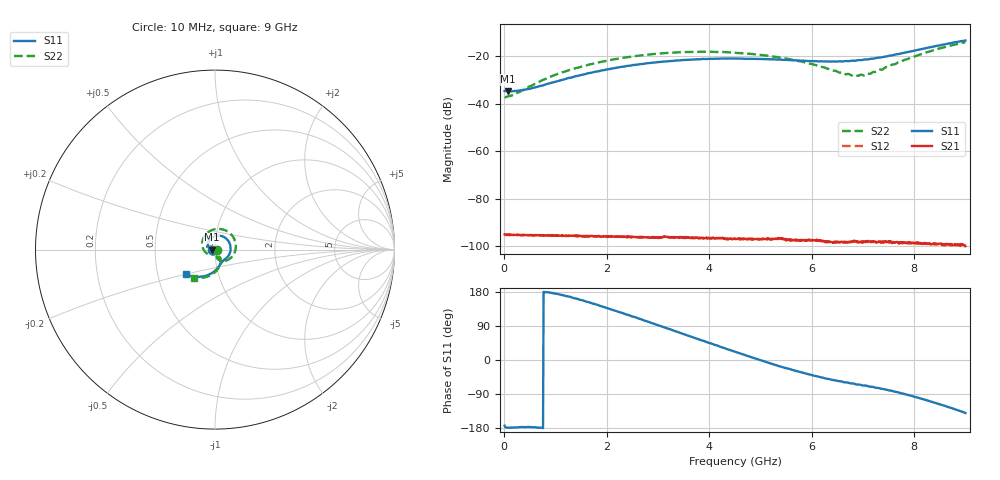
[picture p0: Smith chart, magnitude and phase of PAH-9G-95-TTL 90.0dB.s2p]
! MTS Systemtechnik GmbH
! S-Parameters
! Model: PAH-9G/95-TTL
! Attenuation Step: 90.0dB
#  HZ  S  DB  R  50.00
! Rohde & Schwarz Vector Network Analyzer
! Rohde-Schwarz,ZNB20-2Port,1334333062101652,3.45
! Created: UTC 1/26/2024, 7:42:12 AM
! freq[Hz]  db:S11  ang:S11  db:S21  ang:S21  db:S12  ang:S12  db:S22  ang:S22
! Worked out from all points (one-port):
!   900 points, 10 MHz to 9 GHz, reference 50 ohm
!   lowest |S11| = -34.8 dB at 80 MHz (marker M1), VSWR 1.04, Z = 48.2 - j0.0419 ohm
!   |S11| at or under -10 dB: start of sweep to end of sweep
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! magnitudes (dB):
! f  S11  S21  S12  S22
! 10 MHz  -34.7  -95.0  -95.2  -37.2
! 80 MHz  -34.8  -95.3  -95.2  -36.9
! 170 MHz  -34.8  -95.3  -95.4  -36.4
! 380 MHz  -34.3  -95.2  -95.3  -34.1
! 910 MHz  -31.3  -95.5  -95.5  -28.6
! 1.19 GHz  -29.7  -95.6  -95.7  -26.4
! 1.51 GHz  -27.9  -95.8  -95.9  -24.4
! 2.14 GHz  -25.1  -96.0  -96.1  -21.3
! 3.01 GHz  -22.5  -96.6  -96.6  -18.9
! 3.77 GHz  -21.3  -96.4  -96.4  -18.2
! 4.51 GHz  -21.1  -96.8  -96.9  -18.5
! 5.31 GHz  -21.5  -96.9  -97.1  -20.3
! 5.67 GHz  -21.8  -97.3  -97.5  -21.7
! 6.01 GHz  -22.1  -97.5  -97.6  -23.4
! 6.66 GHz  -22.1  -98.2  -98.7  -27.6
! 6.9 GHz  -21.7  -98.3  -98.1  -28.3
! 7.14 GHz  -21.2  -98.1  -97.9  -27.5
! 7.51 GHz  -19.8  -97.9  -98.0  -24.4
! 7.82 GHz  -18.6  -98.5  -98.4  -21.5
! 8.22 GHz  -16.7  -99.0  -98.9  -18.6
! 8.6 GHz  -15.1  -99.2  -99.2  -16.2
! 9 GHz  -13.4  -100.0  -99.7  -14.2
